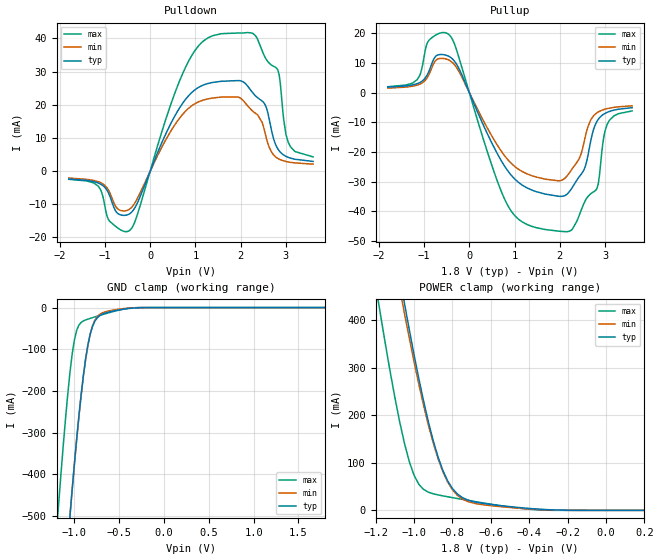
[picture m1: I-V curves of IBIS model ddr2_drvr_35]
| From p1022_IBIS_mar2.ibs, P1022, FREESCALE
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| * P1022 DDR2 Driver Model - 35 Ohm Setting *
[Model]   ddr2_drvr_35
Model_type I/O
Polarity   Non-Inverting
Vinl = 0.7V
Vinh = 1.1V
Vmeas = 0.9V
Cref = 0
Rref = 50
Vref = 0.9V
|   typ   min   max
C_comp   3.628490e-12   2.023040e-12   4.796400e-12
|   typ   min   max
[Voltage range]   1.8V   1.7V   1.9V
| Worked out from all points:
|   slope of the pulldown table from 0 to 0.27 V, typ, clamps not added: 30 ohm
|   slope of the pullup table from 0 to 0.27 V, typ, clamps not added: 28.1 ohm
|   GND clamp passes 1 mA (typ) near -0.33 V on its own axis
|   POWER clamp passes 1 mA (typ) near -0.28 V on its own axis
[Pulldown]
| Warnings regarding non-monotonicity are expected
| Voltage   I(typ)   I(min)   I(max)
-1.8V     -2.402mA   -2.109mA   -2.488mA
-1.15V    -3.582mA   -3.193mA   -4.536mA
-900mV    -7.277mA   -6.325mA   -15.07mA
-725mV    -12.7mA    -11.32mA   -17.09mA
-450mV    -12.85mA   -11.44mA   -17.87mA
750mV     21.06mA    17.6mA     30.39mA
1.575V    27.08mA    22.33mA    41.45mA
2.325V    22.71mA    17.44mA    40.85mA
2.55V     19.72mA    10.83mA    34.03mA
2.825V    6.589mA    3.773mA    30.37mA
3.05V     4.136mA    2.747mA    8.679mA
3.6V      2.906mA    2.078mA    4.268mA
[GND_clamp]
| Voltage   I(typ)   I(min)   I(max)
-1.8V     -2.78A     -2.734A    -2.433A
-1.2V     -918.5mA   -909.4mA   -538.8mA
-1.175V   -846mA     -838.3mA   -467.5mA
-1.1V     -634.6mA   -630.8mA   -267.7mA
-1.05V    -500.5mA   -498.8mA   -155.7mA
-975mV    -315.3mA   -316.1mA   -54.58mA
-900mV    -162.7mA   -164.1mA   -32.05mA
-850mV    -90.19mA   -90.35mA   -27.79mA
-800mV    -46.39mA   -44.74mA   -24.31mA
-650mV    -12.83mA   -9.896mA   -14.51mA
-300mV    -558.6uA   -261.1uA   -231.9uA
1.8V      1.714uA    9.547uA    12.62nA
[Pullup]
| Warnings regarding non-monotonicity are expected
| Voltage   I(typ)   I(min)   I(max)
-1.8V     1.811mA    1.486mA    1.948mA
-1.15V    2.992mA    2.492mA    4.356mA
-900mV    6.859mA    5.768mA    17.4mA
-450mV    12.19mA    10.93mA    19.53mA
850mV     -26.36mA   -22.6mA    -38.02mA
1.975V    -34.97mA   -29.76mA   -46.73mA
2.275V    -32.05mA   -25.7mA    -46.11mA
2.525V    -26.34mA   -17.57mA   -37.7mA
2.775V    -11.24mA   -7.424mA   -33.21mA
2.85V     -9.071mA   -6.563mA   -30.82mA
3.05V     -6.654mA   -5.419mA   -10.65mA
3.6V      -5.104mA   -4.468mA   -6.192mA
[POWER_clamp]
| Warnings about POWER_clamp data never reaching
| zero are expected, and this is okay as long as
| the 0V data are around 10uA or less
| Voltage   I(typ)   I(min)   I(max)
-1.8V     2.412A     2.266A     2.142A
-1.2V     797.2mA    753.3mA    475mA
-1.175V   734.5mA    694.6mA    412.6mA
-1.1V     552mA      523.4mA    238.4mA
-1.05V    436.4mA    415mA      141.5mA
-1V       328.1mA    313.2mA    74.16mA
-925mV    186.2mA    179.4mA    38.2mA
-875mV    112.7mA    109.2mA    32.53mA
-825mV    62.3mA     59.8mA     28.63mA
-725mV    22.56mA    19.44mA    21.45mA
-350mV    2.574mA    1.808mA    967.2uA
200mV     0A         0A         0A
|   typ   min   max
[Ramp]
dV/dt_r   0.671145/1.81258E-10   0.595242/2.57621E-10   0.809324/7.70854E-11
dV/dt_f   0.633607/1.94451E-10   0.548057/2.84554E-10   0.776808/7.37799E-11
